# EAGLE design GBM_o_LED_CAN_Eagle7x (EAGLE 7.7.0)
Gleis Belegt Melder mit CAN
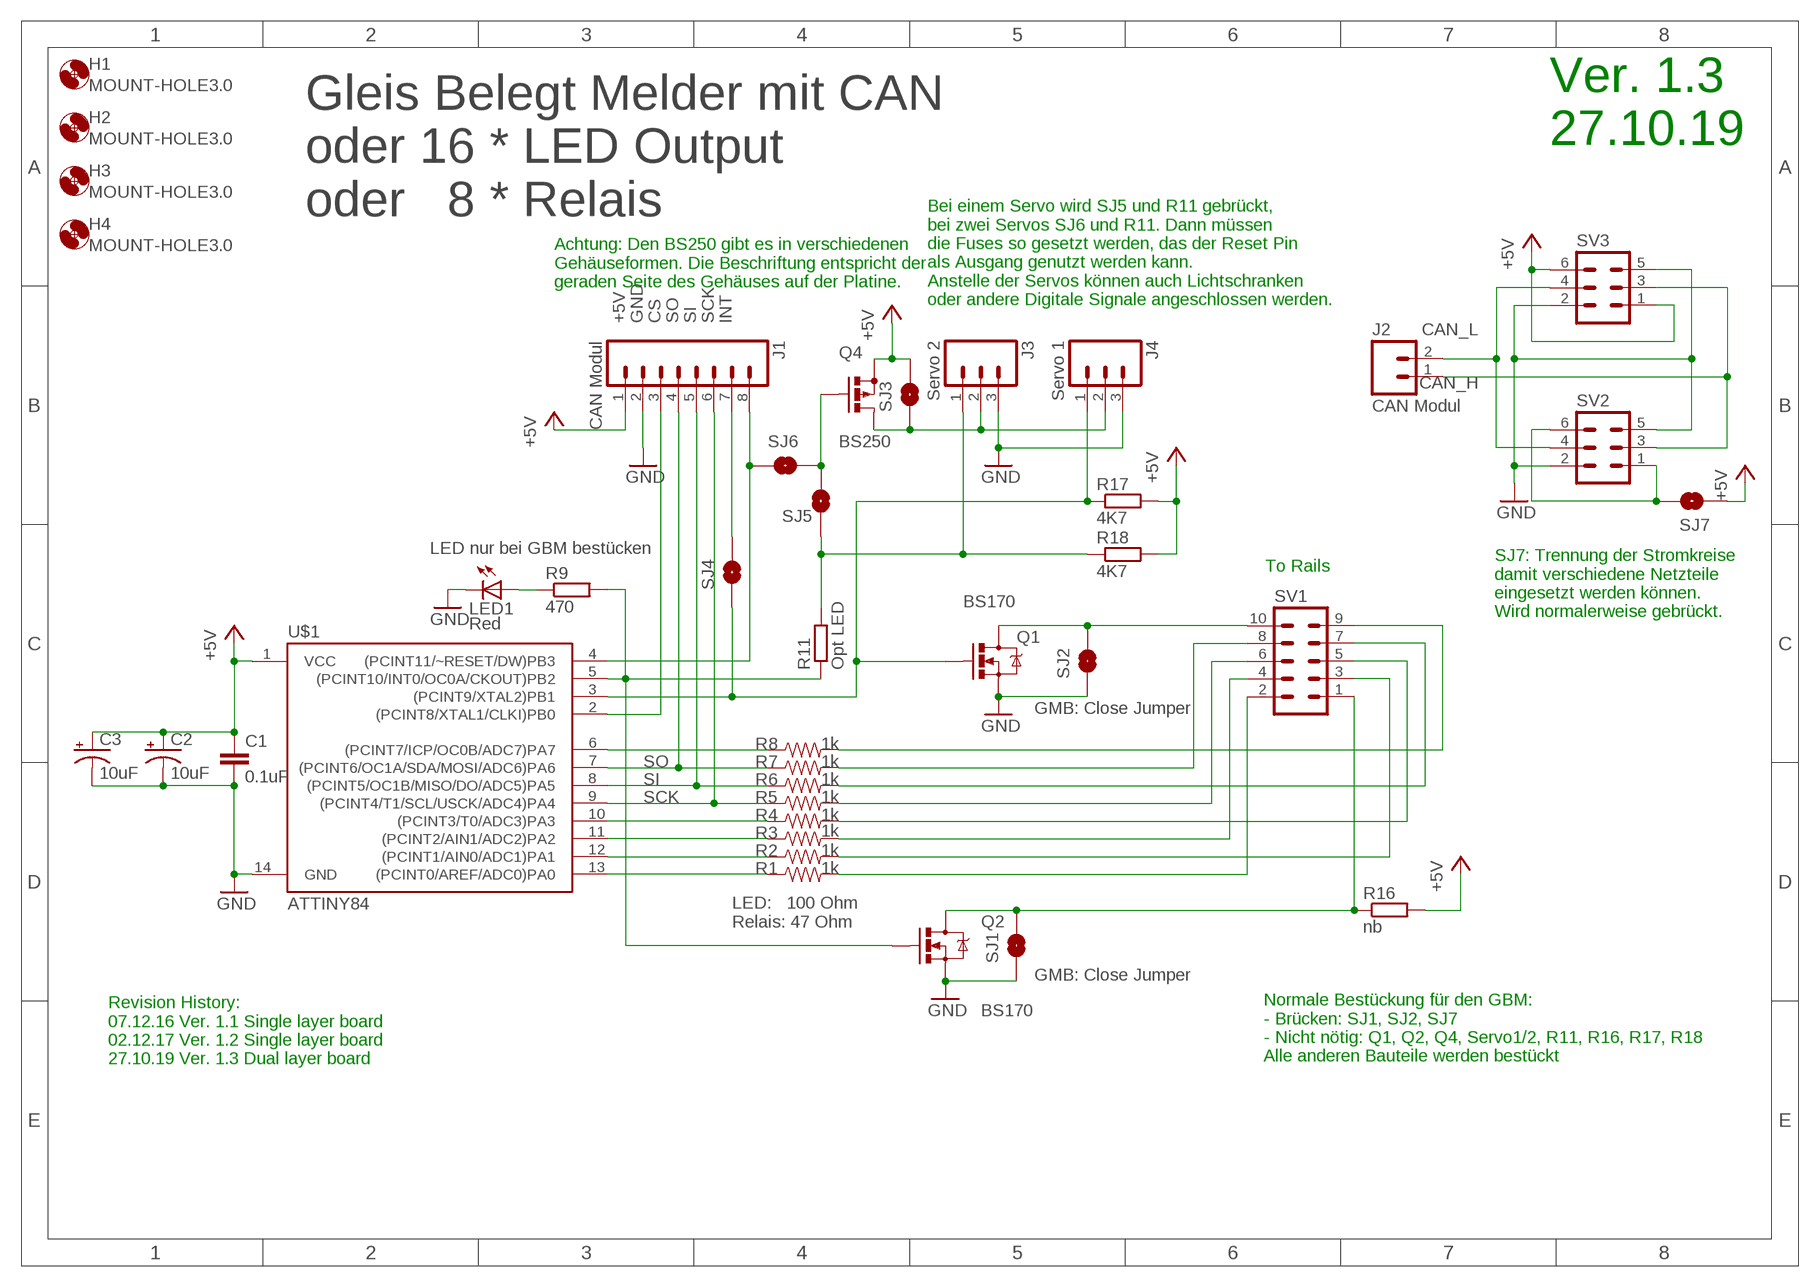
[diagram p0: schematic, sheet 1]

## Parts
C1  0.1uF  0.1UF-50V-20%(PTH)KIT-EZ  [CAP-PTH-SMALL-KIT]
C2  10uF  100UF-25V-20%(PTH)  [CPOL-RADIAL-100UF-25V]
C3  10uF  100UF-25V-20%(PTH)  [CPOL-RADIAL-100UF-25V]
H1  MOUNT-HOLE3.0  [3,0]
H2  MOUNT-HOLE3.0  [3,0]
H3  MOUNT-HOLE3.0  [3,0]
H4  MOUNT-HOLE3.0  [3,0]
J1  CAN Modul  M08  [1X08_ROUND]
J2  CAN Modul  M02PTH3  [1X02_LONGPADS]
J3  Servo 2  M03PTH  [1X03]
J4  Servo 1  M03PTH  [1X03]
LED1  Red  LED3MM  [LED3MM]
Q1  BS170  MOSFET-NCHANNELBS170  [TO-92]
Q2  BS170  MOSFET-NCHANNELBS170  [TO-92]
Q4  BS250  [SOT54E]
R1  1k  1KOHM-1/4W-5%(PTH)  [AXIAL-0.3]
R2  1k  1KOHM-1/4W-5%(PTH)  [AXIAL-0.3]
R3  1k  1KOHM-1/4W-5%(PTH)  [AXIAL-0.3]
R4  1k  1KOHM-1/4W-5%(PTH)  [AXIAL-0.3]
R5  1k  1KOHM-1/4W-5%(PTH)  [AXIAL-0.3]
R6  1k  1KOHM-1/4W-5%(PTH)  [AXIAL-0.3]
R7  1k  1KOHM-1/4W-5%(PTH)  [AXIAL-0.3]
R8  1k  1KOHM-1/4W-5%(PTH)  [AXIAL-0.3]
R9  470  R-EU_0204/7  [0204/7]
R11  Opt LED  R-EU_0204/7  [0204/7]
R16  nb  R-EU_0204/7  [0204/7]
R17  4K7  R-EU_0204/2V  [0204V]
R18  4K7  R-EU_0204/2V  [0204V]
SJ1  SOLDERJUMPERNO  [SJ_2S-NO]
SJ2  SOLDERJUMPERNO  [SJ_2S-NO]
SJ3  SOLDERJUMPERNO  [SJ_2S-NO]
SJ4  SOLDERJUMPERNO  [SJ_2S-NO]
SJ5  SOLDERJUMPERNO  [SJ_2S-NO]
SJ6  SOLDERJUMPERNO  [SJ_2S-NO]
SJ7  SOLDERJUMPERNO  [SJ_2S-NO]
SV1  ML10  [ML10]
SV2  ML6  [ML6]
SV3  ML6  [ML6]
U$1  ATTINY84  ATTINY84ATTINY84-20PU  [DIL14]

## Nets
+5V: C1.1 C2.1(+) C3.1(+) J1.1 Q4.S R16.2 R17.2 R18.2 SJ3.2 SJ7.1 SV3.1 SV3.6 U$1.1(VCC)
CAN_H: J2.1 SV2.3 SV3.3
CAN_L: J2.2 SV2.4 SV3.4
CS: J1.3 U$1.2((PCINT8/XTAL1/CLKI)PB0)
GND: C1.2 C2.2(-) C3.2(-) J1.2 J3.3 J4.3 LED1.K(C) Q1.3(S) Q2.3(S) SJ1.1 SJ2.1 SV2.2 SV2.5 SV3.2 SV3.5 U$1.14(GND)
INT: J1.7 SJ4.2
N$1: R1.P$1 U$1.13((PCINT0/AREF/ADC0)PA0)
N$2: R2.P$1 U$1.12((PCINT1/AIN0/ADC1)PA1)
N$3: R3.P$1 U$1.11((PCINT2/AIN1/ADC2)PA2)
N$4: R4.P$1 U$1.10((PCINT3/T0/ADC3)PA3)
N$5: R8.P$1 U$1.6((PCINT7/ICP/OC0B/ADC7)PA7)
N$6: J4.1 Q1.2(G) R17.1 SJ4.1 U$1.3((PCINT9/XTAL2)PB1)
N$7: J3.1 R11.2 R18.1 SJ5.2
N$8: R1.P$2 SV1.2
N$9: Q2.2(G) R9.2 R11.1 U$1.5((PCINT10/INT0/OC0A/CKOUT)PB2)
N$10: R3.P$2 SV1.4
N$11: R2.P$2 SV1.3
N$12: R5.P$2 SV1.6
N$13: R6.P$2 SV1.7
N$14: R7.P$2 SV1.8
N$15: R8.P$2 SV1.9
N$16: LED1.A R9.1
N$17: SJ7.2 SV2.1 SV2.6
N$18: R4.P$2 SV1.5
N$19: Q2.1(D) R16.1 SJ1.2 SV1.1
N$20: Q1.1(D) SJ2.2 SV1.10
N$23: Q4.G SJ5.1 SJ6.2
N$24: J3.2 J4.2 Q4.D SJ3.1
RESET: J1.8 SJ6.1 U$1.4((PCINT11/~RESET/DW)PB3)
SCK: J1.6 R5.P$1 U$1.9((PCINT4/T1/SCL/USCK/ADC4)PA4)
SI: J1.5 R6.P$1 U$1.8((PCINT5/OC1B/MISO/DO/ADC5)PA5)
SO: J1.4 R7.P$1 U$1.7((PCINT6/OC1A/SDA/MOSI/ADC6)PA6)

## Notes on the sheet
- Ver. 1.3
  27.10.19
- Gleis Belegt Melder mit CAN
  oder 16 * LED Output
  oder   8 * Relais
- Achtung: Den BS250 gibt es in verschiedenen
  Gehäuseformen. Die Beschriftung entspricht der
  geraden Seite des Gehäuses auf der Platine.
- Bei einem Servo wird SJ5 und R11 gebrückt, 
  bei zwei Servos SJ6 und R11. Dann müssen
  die Fuses so gesetzt werden, das der Reset Pin
  als Ausgang genutzt werden kann.
  Anstelle der Servos können auch Lichtschranken
  oder andere Digitale Signale angeschlossen werden.
- SJ7: Trennung der Stromkreise
  damit verschiedene Netzteile
  eingesetzt werden können.
  Wird normalerweise gebrückt.
- LED nur bei GBM bestücken
- To Rails
- GMB: Close Jumper
- LED:   100 Ohm
  Relais: 47 Ohm
- GMB: Close Jumper
- Normale Bestückung für den GBM:
  - Brücken: SJ1, SJ2, SJ7
  - Nicht nötig: Q1, Q2, Q4, Servo1/2, R11, R16, R17, R18
  Alle anderen Bauteile werden bestückt
- Revision History:
  07.12.16 Ver. 1.1 Single layer board 
  02.12.17 Ver. 1.2 Single layer board 
  27.10.19 Ver. 1.3 Dual layer board

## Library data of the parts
C1 = SparkFun-Capacitors:0.1UF-50V-20%(PTH): CAP-08370; PROD_ID: CAP-08370
C2 C3 = SparkFun-Capacitors:100UF-25V-20%(PTH): CAP-08439; PROD_ID: CAP-08439
H1-H4 = holes:MOUNT-HOLE: MOUNTING HOLE with drill center marker
J1 = SparkFun-Connectors:M08: Header 8 Standard 8-pin 0.1" header. Use with straight break away headers (SKU : PRT-00116), right angle break away headers (PRT-00553), swiss pins (PRT-00743), machine pins (PRT-00117), and female headers (PRT-00115).; PROD_ID: CONN-08437
J2 = SparkFun-Connectors:M02: Standard 2-pin 0.1" header. Use with
J3 J4 = SparkFun-Connectors:M03: Header 3 Standard 3-pin 0.1" header. Use with straight break away headers (SKU : PRT-00116), right angle break away headers (PRT-00553), swiss pins (PRT-00743), machine pins (PRT-00117), and female headers (PRT-00115). Molex polarized connector foot print use with SKU : PRT-08232 with associated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
LED1 = led:LED: LED
Q1 Q2 = SparkFun-DiscreteSemi:MOSFET-NCHANNEL: Common NMOSFET Parts MFG P/NStore IDProd ID FDD8780TRANS-09984 SI7820DNTRANS-11055 FDS6630AIC-08089 2N7002PWTRANS-11151 FQP30N06L COM-10213TRANS-10060 BSS123LT1GTRANS-08345 BSS138TRANS-00830 BS170 2N7000
Q4 = transistor-small-signal:BS250: P-CHANNEL MOS FET
R1-R8 = SparkFun-Resistors:1KOHM-1/4W-5%(PTH): RES-08380; PROD_ID: RES-08380
R9 R11 R16 = rcl:R-EU_: RESISTOR, European symbol
R17 R18 = resistor:R-EU_: RESISTOR, European symbol
SJ1-SJ7 = SparkFun-Retired:SOLDERJUMPER: Solder Jumper
SV1 = con-harting-ml:ML10: HARTING; OC_FARNELL: unknown; OC_NEWARK: unknown
SV2 SV3 = con-harting-ml:ML6: HARTING; OC_FARNELL: unknown; OC_NEWARK: unknown
U$1 = SparkFun-DigitalIC:ATTINY84: Atmel 14-pin 2/4/8kB flash uC

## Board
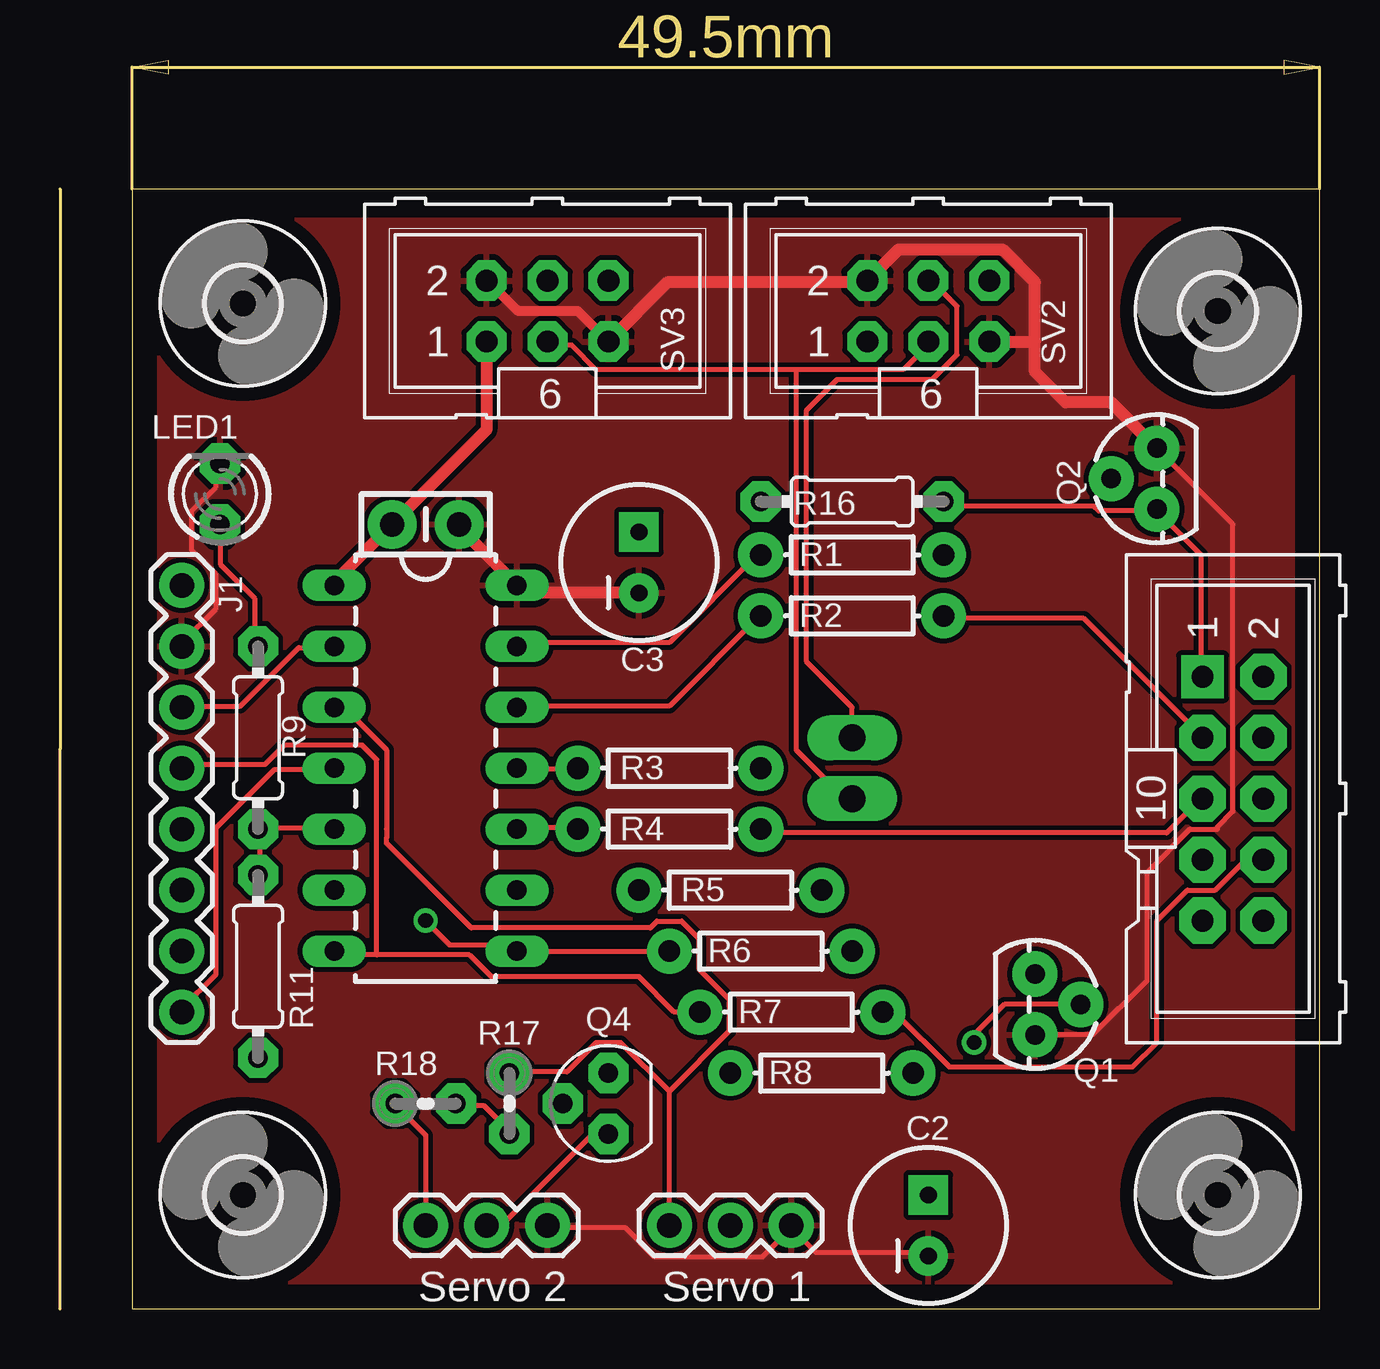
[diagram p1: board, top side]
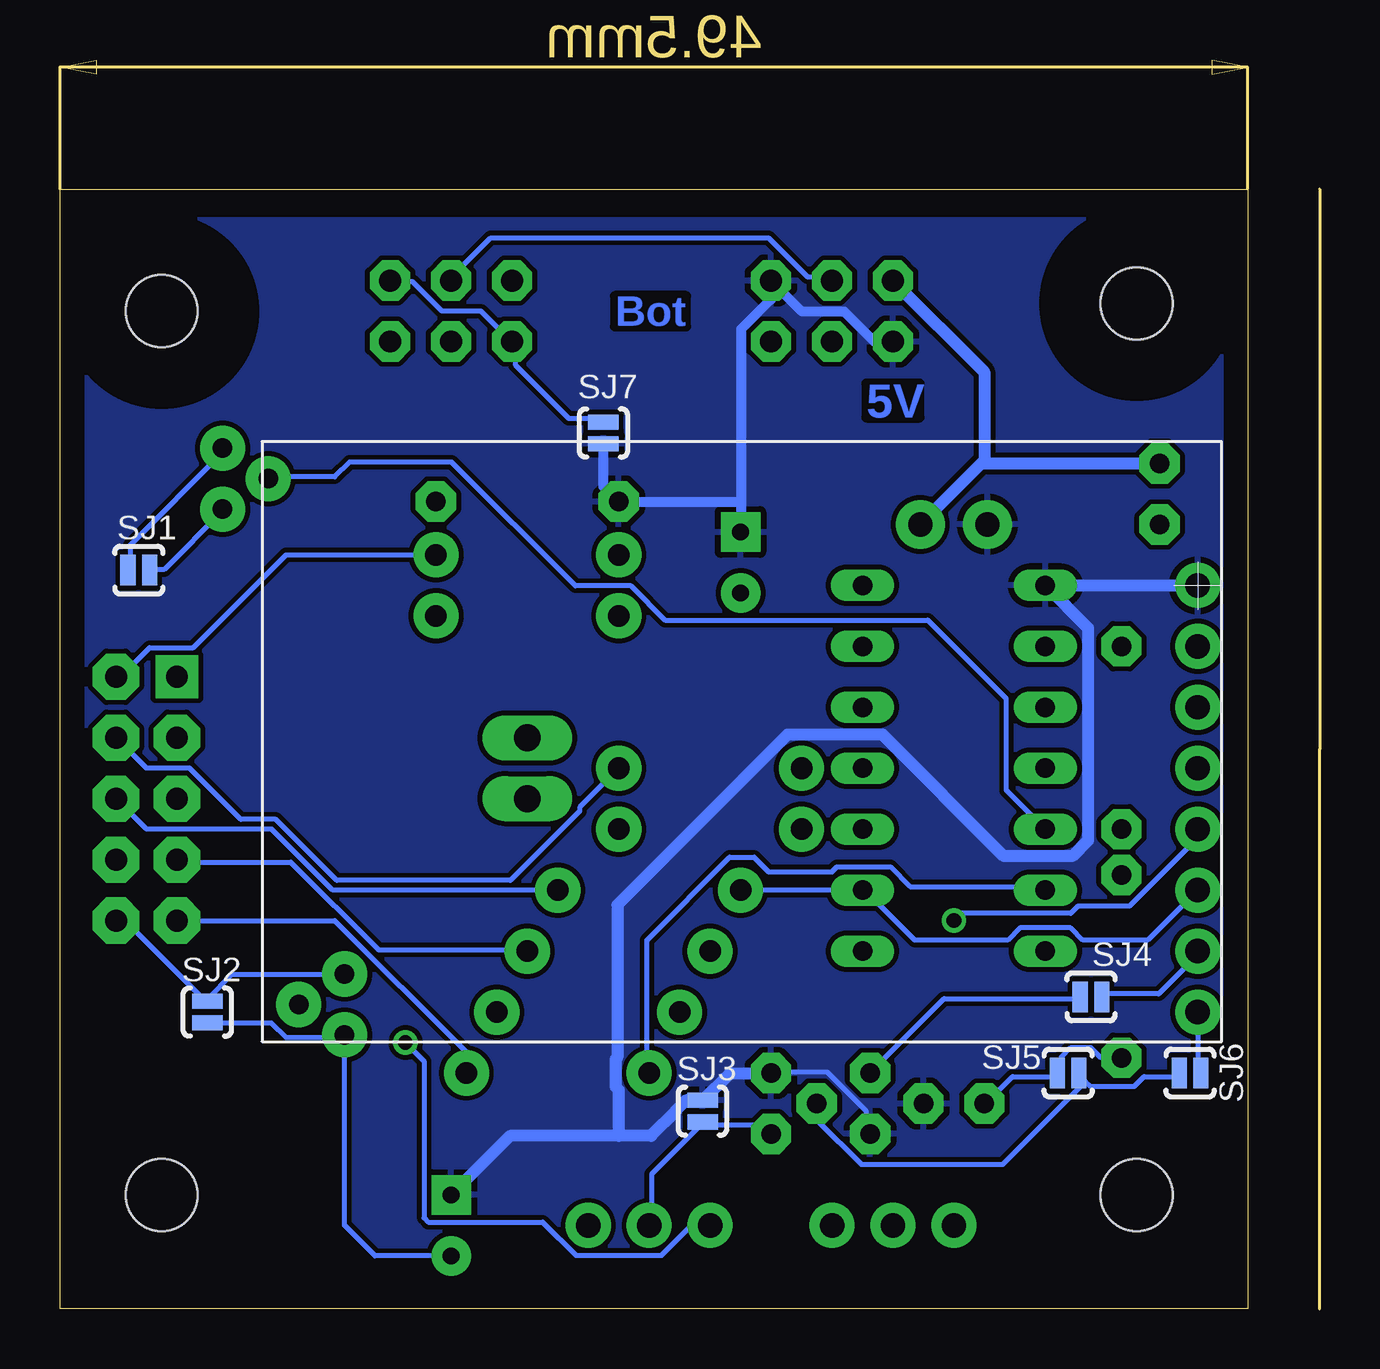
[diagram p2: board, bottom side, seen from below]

Size 52.5 x 52.04 mm. Coordinates in mm from the lower left corner, seen from the top.
Outline: 3,46.66 3,0 52.5,0 52.5,46.66 3,46.66
Copper layers (1*16): Top 0.035mm / dielectric 1.5mm / Bottom 0.035mm
Design rules "default *": minimum track width 8mil, minimum drill 24mil, track to track 8mil, track to pad 8mil, pad to pad 8mil, via to via 8mil, smd to smd 8mil, copper to edge 40mil, drill to drill 8mil, minimum pad ring 10mil, minimum via ring 8mil, stop-mask expansion 4mil, vias tented up to drill 0mil, thermal gap 10mil

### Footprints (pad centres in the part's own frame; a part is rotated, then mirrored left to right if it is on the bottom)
CAP-PTH-SMALL-KIT = drill 1.016 pad 2.032: 1 -1.397,0; 2 1.397,0
CPOL-RADIAL-100UF-25V = drill 0.7 pad 1.651 square: 1 1.27,0 | drill 0.7 pad 1.651: 2 -1.27,0
3,0 = hole 3: 0,0
1X08_ROUND = drill 1.016 pad 1.88: 1 0,0; 2 2.54,0; 3 5.08,0; 4 7.62,0; 5 10.16,0; 6 12.7,0; 7 15.24,0; 8 17.78,0
1X02_LONGPADS = drill 1.118 pad 1.88 long: 1 0,0; 2 2.54,0
1X03 = drill 1.016 pad 1.88: 1 0,0; 2 2.54,0; 3 5.08,0
LED3MM = drill 0.813 pad 1.676 octagon: A -1.27,0; K 1.27,0
TO-92 = drill 0.813 pad 1.88: 1 -1.27,0; 2 0,1.905; 3 1.27,0
SOT54E = drill 0.813 pad 1.676 octagon: D -1.27,0; G 0,1.905; S 1.27,0
AXIAL-0.3 = drill 0.9 pad 1.88: P$1 -3.81,0; P$2 3.81,0
0204/7 = drill 0.813 pad 1.676 octagon: 1 -3.81,0; 2 3.81,0
0204V = drill 0.813 pad 1.676 octagon: 1 -1.27,0; 2 1.27,0
SJ_2S-NO = smd 0.635 x 1.27: 1 -0.45,0; 2 0.45,0
ML10 = drill 0.914 pad 1.778 square: 1 -5.08,-1.27 | drill 0.914 pad 1.93 octagon: 2 -5.08,1.27; 3 -2.54,-1.27; 4 -2.54,1.27; 5 0,-1.27; 6 0,1.27; 7 2.54,-1.27; 8 2.54,1.27; 9 5.08,-1.27; 10 5.08,1.27
ML6 = drill 0.914 pad 1.676 octagon: 1 -2.54,-1.27; 2 -2.54,1.27; 3 0,-1.27; 4 0,1.27; 5 2.54,-1.27; 6 2.54,1.27
DIL14 = drill 0.813 long: 1 -8.89,-3.81; 2 -6.35,-3.81; 3 -3.81,-3.81; 4 -1.27,-3.81; 5 1.27,-3.81; 6 3.81,-3.81; 7 6.35,-3.81; 8 6.35,3.81; 9 3.81,3.81; 10 1.27,3.81; 11 -1.27,3.81; 12 -3.81,3.81; 13 -6.35,3.81; 14 -8.89,3.81

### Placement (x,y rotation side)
C1  15.24,32.69 0 top
C2  36.2,3.48 90 top
C3  24.13,31.1 90 top
H1  7.62,4.75 270 top
H2  48.26,41.58 270 top
H3  7.62,41.9 270 top
H4  48.26,4.75 270 top
J1  5.08,30.15 270 top
J2  33.02,21.26 90 top
J3  15.24,3.48 0 top
J4  25.4,3.48 0 top
LED1  6.67,33.96 90 top
Q1  40.64,12.69 270 top
Q2  45.72,34.59 90 top
Q4  22.86,8.56 90 top
R1  33.02,31.42 0 top
R2  33.02,28.88 0 top
R3  25.4,22.53 0 top
R4  25.4,19.99 0 top
R5  27.94,17.45 0 top
R6  29.21,14.91 0 top
R7  30.48,12.37 0 top
R8  31.75,9.83 0 top
R9  8.26,23.8 270 top
R11  8.26,14.28 270 top
R16  33.02,33.64 180 top
R17  18.73,8.56 270 top
R18  15.24,8.56 0 top
SJ1  49.21,30.79 0 bottom
SJ2  46.35,12.37 90 bottom
SJ3  25.72,8.24 90 bottom
SJ4  9.53,13 0 bottom
SJ5  10.48,9.83 180 bottom
SJ6  5.4,9.83 180 bottom
SJ7  29.84,36.5 90 bottom
SV1  48.9,21.26 270 top
SV2  36.2,41.58 0 top
SV3  20.32,41.58 0 top
U$1  15.24,21.26 270 top

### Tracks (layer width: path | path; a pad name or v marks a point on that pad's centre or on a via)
+5V
  Top 0.203: R18.2 16.66,8.46 17.68,8.46 18.69,7.44 R17.2
  Top 0.508: U$1.1 11.43,30.28 C1.1 17.78,36.63 SV3.1
  Bottom 0.203: 27.86,7.21 26.42,8.66 25.81,8.66 SJ3.2 | R17.2 18.9,7.44 18.9,8.26 20.52,9.88 22.76,9.88 Q4.S
  Bottom 0.406: SV3.1 18.56,40.31 19.8,41.55 21.57,41.55 SV3.6 22.86,42.07 24.11,40.83 24.11,33.64 | C3.1 24.11,32.4 24.11,33.64 | SJ7.1 29.84,34.28 R16.2 24.11,33.64
  Bottom 0.508: J1.1 U$1.1 9.65,28.37 9.65,19.53 10.31,18.87 13.15,18.87 18.21,23.93 22.17,23.93 29.26,16.84 29.26,10.48 29.34,10.41 29.34,9.25 29.21,9.12 29.21,7.21 | 29.21,7.21 27.86,7.21 26.81,8.27 26.81,8.3 26.42,8.69 SJ3.2 24.58,9.83 Q4.S | 29.21,7.21 33.73,7.21 C2.1
  pour Bottom: 3.81,45.39 52.07,45.39 52.07,0.94 5.08,0.94 3.81,2.21
CAN_H
  Top 0.203: 30.68,39.14 35.15,39.14 36.17,40.16 SV2.3 | 30.68,39.14 22.35,39.14 21.34,40.16 20.32,40.16 SV3.3 | 30.68,39.14 30.68,23.29 32.72,21.26 J2.1
CAN_L
  Top 0.203: SV2.4 36.37,42.8 37.39,41.78 37.39,39.75 36.37,38.73 32.4,38.73 31.11,37.45 31.11,26.98 33.02,25.07 J2.2
  Bottom 0.203: SV3.4 20.32,43 21.34,43 22.96,44.63 34.54,44.63 36.17,43 SV2.4
CS
  Top 0.203: U$1.2 11.38,27.56 9.96,27.56 7.52,25.12 5.08,25.12 J1.3
GND
  Top 0.203: 30.48,3.38 31.5,2.36 36.17,2.36 C2.2 | 30.48,3.38 29.26,2.16 24.79,2.16 23.57,3.38 20.32,3.38 J3.3 | 30.48,3.38 J4.3 | LED1.K 6.5,35.08 6.5,34.27 5.49,33.25 5.49,31.62 6.5,30.61 6.5,29.19 5.08,27.76 J1.2 | 33.53,42.8 SV2.2 | Q1.3 40.66,11.44 43.06,11.44 45.31,13.7 45.31,18.21 47.1,19.99 48.26,19.99 48.26,20.1 48.9,20.73 48.9,32.69 Q2.3
  Top 0.406: SV3.5 21.59,41.58 19.1,41.58 17.83,42.85 SV3.2
  Top 0.508: SV3.5 25.35,42.8 33.53,42.8 33.6,42.8 34.95,44.14 39.27,44.14 40.64,42.78 40.64,40.31 | Q2.3 43.81,37.77 41.91,37.77 40.64,39.04 40.64,40.31 | SV2.5 40.64,40.31 | C3.2 19.37,29.83 U$1.14 16.64,32.56 C1.2
  Bottom 0.203: 40.64,11.3 43.08,11.3 43.69,11.91 46.33,11.91 SJ2.1 | 40.64,11.3 Q1.3 | SJ1.1 49.58,30.81 49.58,31.83 45.72,35.69 Q2.3 | C2.2 39.37,2.21 40.64,3.48 40.64,11.3
  Bottom 0.508: C1.2 14.1,35.23 13.97,35.23 | 13.97,35.23 LED1.K | SV3.2 13.97,39.04 13.97,35.23
  pour Top: 3.81,45.39 52.07,45.39 52.07,0.94 3.81,0.94
INT
  Bottom 0.203: SJ4.2 8.94,13.13 6.71,13.13 5.08,14.76 J1.7
N$1
  Top 0.203: U$1.13 19.1,27.76 25.4,27.76 29.06,31.42 R1.P$1
N$2
  Top 0.203: U$1.12 19.1,25.12 25.4,25.12 29.06,28.78 R2.P$1
N$3
  Top 0.203: U$1.11 19.1,22.48 21.54,22.48 R3.P$1
N$4
  Top 0.203: U$1.10 19.1,20.04 21.54,20.04 R4.P$1
N$5
  Bottom 0.203: U$1.6 11.58,17.6 17.07,17.6 17.88,18.42 20.12,18.42 20.32,18.21 22.96,18.21 23.57,18.82 24.59,18.82 28.04,15.37 28.04,9.88 R8.P$1
N$6  (via drill 0.61)
  Top 0.203: J4.1 25.4,9.07 | U$1.3 11.58,24.92 11.99,24.92 13.61,23.29 13.61,19.99 13.61,19.62 13.61,19.4 17.14,15.88 24.61,15.88 24.88,16.16 25.92,16.16 26.64,15.43 26.64,14.16 27.91,12.89 27.91,11.58 25.4,9.07 | 25.4,9.07 23.37,11.1 22.35,11.1 21.13,9.88 18.9,9.88 R17.1 | Q1.2 39.37,12.69 38.1,11.42 v38.1,11.1
  Bottom 0.203: SJ4.1 10.16,12.93 15.65,12.93 18.69,9.88 R17.1 | J4.1 26.18,3.48 27.42,2.23 31,2.23 32.38,3.62 37.15,3.62 37.33,3.8 37.33,10.32 v38.1,11.1
N$7
  Top 0.203: J3.1 15.24,7.24 14.02,8.46 R18.1
  Bottom 0.203: R18.1 13.82,8.66 12.8,9.68 10.97,9.68 SJ5.2 10.77,9.88 10.77,10.49 10.36,10.9 9.55,10.9 9.14,10.49 8.33,10.49 R11.2
N$8
  Bottom 0.203: R1.P$2 43.08,31.42 46.94,27.56 48.77,27.56 49.99,26.34 SV1.2
N$9
  Top 0.203: U$1.5 11.38,20.04 8.33,20.04 R9.2 8.33,19.84 8.33,18.21 R11.1
  Bottom 0.203: Q2.2 43.69,34.67 41.05,34.67 40.44,35.28 36.17,35.28 31.01,30.12 28.69,30.12 27.27,28.7 16.33,28.7 13.06,25.43 13.06,21.62 U$1.5
N$10
  Bottom 0.203: SV1.4 48.9,22.53 47.1,22.53 44.97,20.4 43.5,20.4 40.96,17.86 33.72,17.86 30.84,20.74 30.84,20.9 R3.P$2
N$11
  Top 0.203: R2.P$2 36.98,28.78 42.67,28.78 47.55,23.9 SV1.3
N$12
  Bottom 0.203: R5.P$2 41.13,17.45 43.67,19.99 48.9,19.99 SV1.6
N$13
  Bottom 0.203: R6.P$2 33.12,14.96 39.22,14.96 42.88,18.62 47.55,18.62 SV1.7
N$14
  Top 0.203: SV1.8 49.42,18.72 48.15,17.45 46.99,17.45 45.72,16.18 45.72,11.1 44.7,10.08 37.07,10.08 34.78,12.37 R7.P$2
N$15
  Bottom 0.203: R8.P$2 35.56,10.69 41.05,16.18 SV1.9
N$16
  Top 0.203: LED1.A 6.71,32.64 6.71,31.01 8.13,29.59 8.13,27.76 R9.1
N$17
  Bottom 0.203: SJ7.2 29.87,37.11 31.29,37.11 33.53,39.34 33.53,40.16 SV2.1 33.73,40.36 34.95,41.58 36.58,41.58 37.8,42.8 38.61,42.8 SV2.6
N$18
  Top 0.203: R4.P$2 29.26,19.84 46.13,19.84 47.55,21.26 SV1.5
N$19
  Top 0.203: 45.72,33.25 43.28,33.25 43.08,33.45 36.98,33.45 R16.1 | 45.72,33.25 47.55,31.42 47.55,26.34 SV1.1 | 45.72,33.25 Q2.1
  Bottom 0.203: SJ1.2 48.56,30.81 48.16,30.81 45.72,33.25 Q2.1
N$20
  Bottom 0.203: SV1.10 49.78,16.18 46.53,12.93 SJ2.2 46.33,12.93 45.31,13.95 40.64,13.95 Q1.1
N$23
  Bottom 0.203: 9.75,9.47 9.96,9.68 SJ5.1 9.75,9.47 | 9.75,9.47 9.55,9.27 7.72,9.27 7.32,9.68 5.89,9.68 SJ6.2 | 9.75,9.47 13.21,6.02 19.1,6.02 20.93,7.85 20.93,8.46 Q4.G
N$24
  Top 0.203: J3.2 17.88,3.58 18.49,3.58 22.15,7.24 22.76,7.24 Q4.D
  Bottom 0.203: Q4.D 22.96,7.44 23.16,7.65 25.6,7.65 SJ3.1 25.81,7.65 27.84,5.61 27.84,3.58 J4.2
RESET
  Top 0.203: U$1.4 11.38,22.48 8.94,22.48 6.5,20.04 6.5,13.95 5.08,12.52 J1.8
  Bottom 0.203: J1.8 5.08,9.88 SJ6.1
SCK
  Bottom 0.203: R5.P$1 U$1.9 18.9,17.4 16.87,15.37 13,15.37 12.49,15.88 10.37,15.88 9.86,15.37 7.16,15.37 J1.6
SI  (via drill 0.61)
  Top 0.203: v15.24,16.18 16.26,15.16 18.8,15.16 U$1.8 R6.P$1
  Bottom 0.203: J1.5 5.08,19.63 7.92,16.79 10.06,16.79 10.37,16.48 14.94,16.48 v15.24,16.18
SO
  Top 0.203: 13.21,14.76 17.07,14.76 17.98,13.84 24.13,13.84 25.6,12.37 R7.P$1 | 13.21,14.76 11.58,14.76 U$1.7 | 13.21,14.76 13.21,22.89 12.6,23.5 9.35,23.5 8.53,22.68 5.08,22.68 J1.4

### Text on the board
Bottom: Bot | 5V
tDocu: 5V & CAN | C1 0.1uF | + | CAN L | CAN H | GBM/LED CAN / Luisa & Hardi | Ver. 1.3 | 31.10.19 | Brown | Brown

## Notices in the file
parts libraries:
SparkFun-DigitalIC: Licensing: Creative Commons ShareAlike 4.0 International - https://creativecommons.org/licenses/by-sa/4.0
